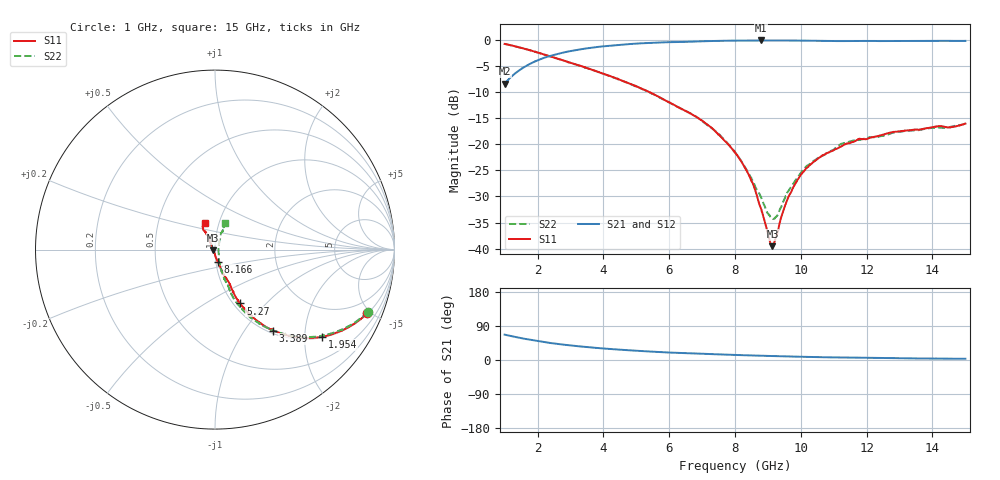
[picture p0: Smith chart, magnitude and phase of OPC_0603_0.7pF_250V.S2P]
! FILE NAME
! DATE 08/21/2012  14:33
! CORRECTED  DATA
# GHz  S  MA  R  50.00
!  FREQ  S11M  S11A  S21M  S21A  S12M  S12A  S22M  S22A
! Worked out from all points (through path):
!   1601 points, 1 GHz to 15 GHz, reference 50 ohm
!   highest |S21| = -0.07 dB at 8.796 GHz (marker M1); lowest = -8.4 dB at 1 GHz (marker M2)
!   lowest |S11| = -39.5 dB at 9.137 GHz (marker M3), VSWR 1.02, Z = 49 - j0.364 ohm
!   |S11| at or under -10 dB: 5.402 GHz to end of sweep
!   |S22| runs from -34.3 to -0.7 dB; largest |S21 - S12| = 0.0083
!   S11 on the Smith chart (normalised r, x): 1 GHz: 1.04, -4.77; 1.954 GHz: 1.03, -2.43; 3.389 GHz: 1.04, -1.36; 5.27 GHz: 1.07, -0.72; 8.166 GHz: 1.02, -0.14; 15 GHz: 0.86, +0.26
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1  0.9196 -22.7  0.3823 67.0  0.382 67.0  0.9192 -22.3
1.95375  0.7687 -39.2  0.6302 50.7  0.6297 50.7  0.7687 -38.5
3.33625  0.5622 -53.9  0.8181 35.5  0.8176 35.5  0.5601 -53.9
3.38875  0.5553 -54.5  0.8233 35.0  0.8233 35.0  0.5532 -54.4
5.27  0.3312 -64.9  0.9358 23.1  0.9351 23.1  0.3296 -67.3
5.6725  0.2869 -66.5  0.9491 21.2  0.9489 21.1  0.2856 -69.4
7.0375  0.1656 -69.3  0.975 16.4  0.975 16.4  0.1643 -72.5
7.51  0.1237 -72.0  0.9827 14.9  0.9823 14.9  0.1256 -72.9
8  0.08335 -75.3  0.988 13.4  0.9872 13.4  0.0842 -72.6
8.16625  0.07038 -77.1  0.9883 12.9  0.9885 12.9  0.07116 -70.7
8.53375  0.04262 -84.1  0.9899 12.0  0.9889 12.0  0.04514 -61.4
8.79625  0.02387 -91.6  0.9919 11.3  0.991 11.3  0.03084 -48.1
9.05  0.01202 -130.3  0.9906 10.6  0.9893 10.7  0.02077 -17.6
9.1375  0.01056 -159.4  0.9904 10.4  0.9901 10.5  0.01943 -1.8
9.28625  0.01395 157.3  0.9904 10.2  0.99 10.2  0.02078 23.7
9.4525  0.02221 138.3  0.9908 9.8  0.9901 9.8  0.02754 43.7
9.65375  0.03258 128.7  0.9908 9.3  0.9904 9.3  0.03698 53.8
9.9775  0.04985 123.6  0.989 8.6  0.9889 8.6  0.05212 62.9
10.33625  0.06571 119.4  0.9873 7.9  0.9864 7.9  0.06738 65.0
11.255  0.09639 119.1  0.9788 6.7  0.9786 6.7  0.102 68.9
12.6725  0.1286 120.7  0.9771 5.1  0.9769 5.1  0.1251 70.0
15  0.1583 111.1  0.9831 3.3  0.9824 3.3  0.1584 69.7
